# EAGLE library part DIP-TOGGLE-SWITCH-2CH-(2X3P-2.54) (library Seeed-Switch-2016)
311010004
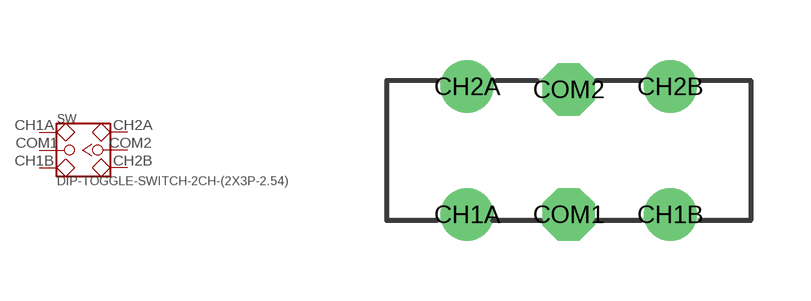
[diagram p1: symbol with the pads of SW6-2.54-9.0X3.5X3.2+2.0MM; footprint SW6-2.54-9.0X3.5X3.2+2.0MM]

Designator prefix SW

## DIP-TOGGLE-SWITCH-2CH-(2X3P-2.54) (MPN: MS-22D18 G2 ROHS)  [SW6-2.54-9.0X3.5X3.2+2.0MM]
CH1A  CH1A
CH1B  CH1B
CH2A  CH2A
CH2B  CH2B
COM1  COM1
COM2  COM2

## Footprint SW6-2.54-9.0X3.5X3.2+2.0MM (pad centres in mm)
drill 0.813 pad 1.27: CH1A -2.54,-1.6; CH1B 2.54,-1.6; CH2A -2.54,1.6; CH2B 2.54,1.6
drill 0.813 pad 1.27 octagon: COM1 0,-1.6; COM2 0,1.524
